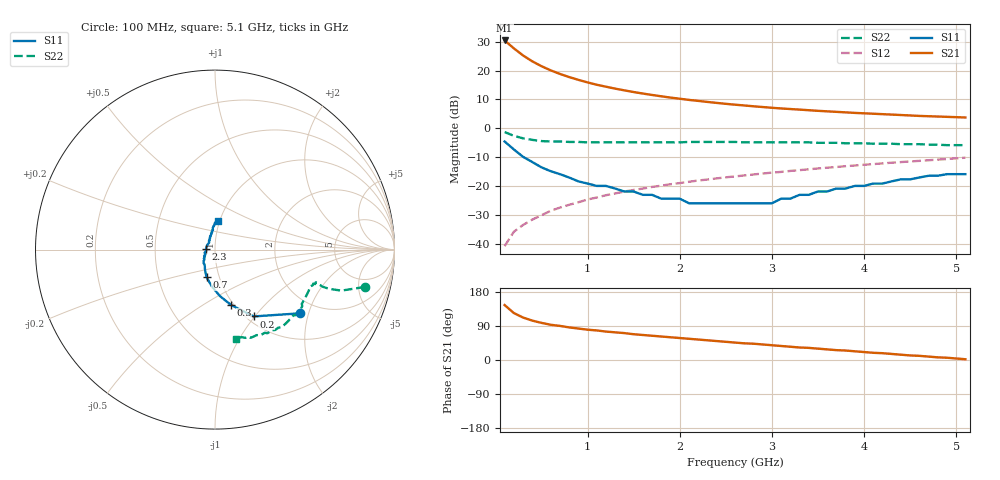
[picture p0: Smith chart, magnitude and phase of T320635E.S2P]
!AT-32063
!S AND NOISE PARAMETERS per side at Vce=5 V  Ic=20mA.  LAST UPDATED 11-11-96
# ghz s ma r 50
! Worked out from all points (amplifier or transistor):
!   51 points, 100 MHz to 5.1 GHz, reference 50 ohm
!   highest |S21| = 30.5 dB at 100 MHz (marker M1)
!   |S21| within 3 dB of that: start of sweep to 210.7 MHz
!   unconditionally stable (mu >= 1): 584.1 MHz to 3.586 GHz
!   at 900 MHz: K = 1.06, MAG = 19.7 dB, |S12| = -25.7 dB
!   at 2.6 GHz: K = 1.04, MAG = 11.2 dB, |S12| = -16.7 dB
!   at 5.1 GHz: K = 0.92, MSG = 7.0 dB, |S12| = -10.2 dB
!   lowest NFmin = 1.50 dB at 900 MHz
!   S11 on the Smith chart (normalised r, x): 100 MHz: 1.61, -1.75; 200 MHz: 1.08, -0.99; 300 MHz: 0.97, -0.66; 700 MHz: 0.87, -0.27; 2.3 GHz: 0.90, +0.00; 5.1 GHz: 0.98, +0.32
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0.1  0.59 -37.0  33.46 145.0  0.009 76.0  0.86 -14.0
0.2  0.43 -60.0  24.42 124.0  0.016 71.0  0.74 -18.0
0.3  0.32 -74.0  18.38 112.0  0.021 70.0  0.67 -19.0
0.4  0.26 -84.0  14.53 104.0  0.026 71.0  0.63 -19.0
0.5  0.21 -94.0  11.96 98.0  0.031 71.0  0.6 -18.0
0.6  0.18 -101.0  10.14 93.0  0.037 72.0  0.59 -18.0
0.7  0.16 -107.0  8.79 90.0  0.042 72.0  0.59 -19.0
0.8  0.14 -112.0  7.75 86.0  0.047 72.0  0.58 -19.0
0.9  0.12 -118.0  6.93 83.0  0.052 72.0  0.58 -20.0
1  0.11 -121.0  6.26 80.0  0.058 72.0  0.57 -21.0
1.1  0.1 -126.0  5.7 78.0  0.063 71.0  0.57 -22.0
1.2  0.1 -129.0  5.27 75.0  0.069 71.0  0.57 -23.0
1.3  0.09 -135.0  4.88 73.0  0.074 70.0  0.57 -24.0
1.5  0.08 -141.0  4.26 68.0  0.085 69.0  0.57 -26.0
1.8  0.06 -153.0  3.59 62.0  0.101 67.0  0.57 -30.0
2.1  0.05 -169.0  3.11 56.0  0.118 64.0  0.58 -33.0
2.3  0.05 177.0  2.87 52.0  0.129 63.0  0.58 -36.0
2.6  0.05 157.0  2.57 46.0  0.146 60.0  0.58 -39.0
3  0.05 131.0  2.27 39.0  0.17 57.0  0.57 -44.0
3.5  0.08 110.0  2.01 30.0  0.201 52.0  0.56 -51.0
4.3  0.12 96.0  1.73 16.0  0.253 43.0  0.54 -62.0
5.1  0.16 85.0  1.54 2.0  0.309 34.0  0.51 -77.0
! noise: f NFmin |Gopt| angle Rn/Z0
0.9  1.5  0.18  71  0.2
1.8  1.78  0.19  147  0.16
2.4  1.96  0.24  -162  0.14
